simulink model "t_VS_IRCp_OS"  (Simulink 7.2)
settings: Solver=ode3  StartTime=0.0  StopTime=0.02  FixedStep=1e-5  RelTol=1e-3

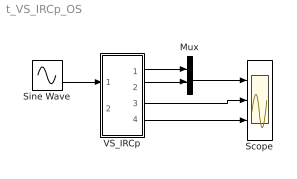
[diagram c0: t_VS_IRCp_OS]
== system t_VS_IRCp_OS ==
  Mux : Mux  Inputs=2
  Scope : Scope  NumInputPorts=3
  Sine Wave : Sin  Amplitude=230*sqrt(2)  Frequency=1000*pi  SampleTime=0
  VS_IRCp : Subsystem  mask(VS_IRCp_OS){R=1, C=100e-6, VC0=0, RCs=1}
      mask prompts: R "Load Resistance"; C "Load Capacitance"; VC0 "Initial Cap Voltage"; RCs "Cap Series Res"
      mask help: Open source VS_IRCp Input Vector: u[0]= Vs, Source Voltage u[1]= IL, Load Current Output Vector: y[0]=IC, Capacitor current y[1]=VC, Capacitor Voltage y[2]=IR, current of Load Resistance y[3]=VRs, Voltage on series Resistance Parameter Vector: p[0]=R1 p[1]=C p[2]=VC0 p[3]=Rs
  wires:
  Sine Wave/1 -> VS_IRCp/1(v)
  VS_IRCp/1(iC) -> Mux/1
  VS_IRCp/2(vC) -> Mux/2
  Mux/1 -> Scope/1
  VS_IRCp/3(vR) -> Scope/2
  VS_IRCp/4(vRS) -> Scope/3

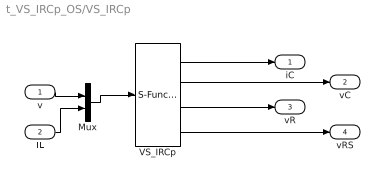
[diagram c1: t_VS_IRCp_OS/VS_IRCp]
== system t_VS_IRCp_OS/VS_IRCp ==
  v : Inport
  IL : Inport  Port=2
  Mux : Mux  Inputs=2
  VS_IRCp : S-Function  FunctionName=s_VS_IRCp_OS  Parameters=[R,C, VC0, RCs]  EnableBusSupport=off
  iC : Outport
  vC : Outport  Port=2
  vR : Outport  Port=3
  vRS : Outport  Port=4
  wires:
  Mux/1 -> VS_IRCp/1
  IL/1 -> Mux/2
  v/1 -> Mux/1
  VS_IRCp/1 -> iC/1
  VS_IRCp/2 -> vC/1
  VS_IRCp/3 -> vR/1
  VS_IRCp/4 -> vRS/1
